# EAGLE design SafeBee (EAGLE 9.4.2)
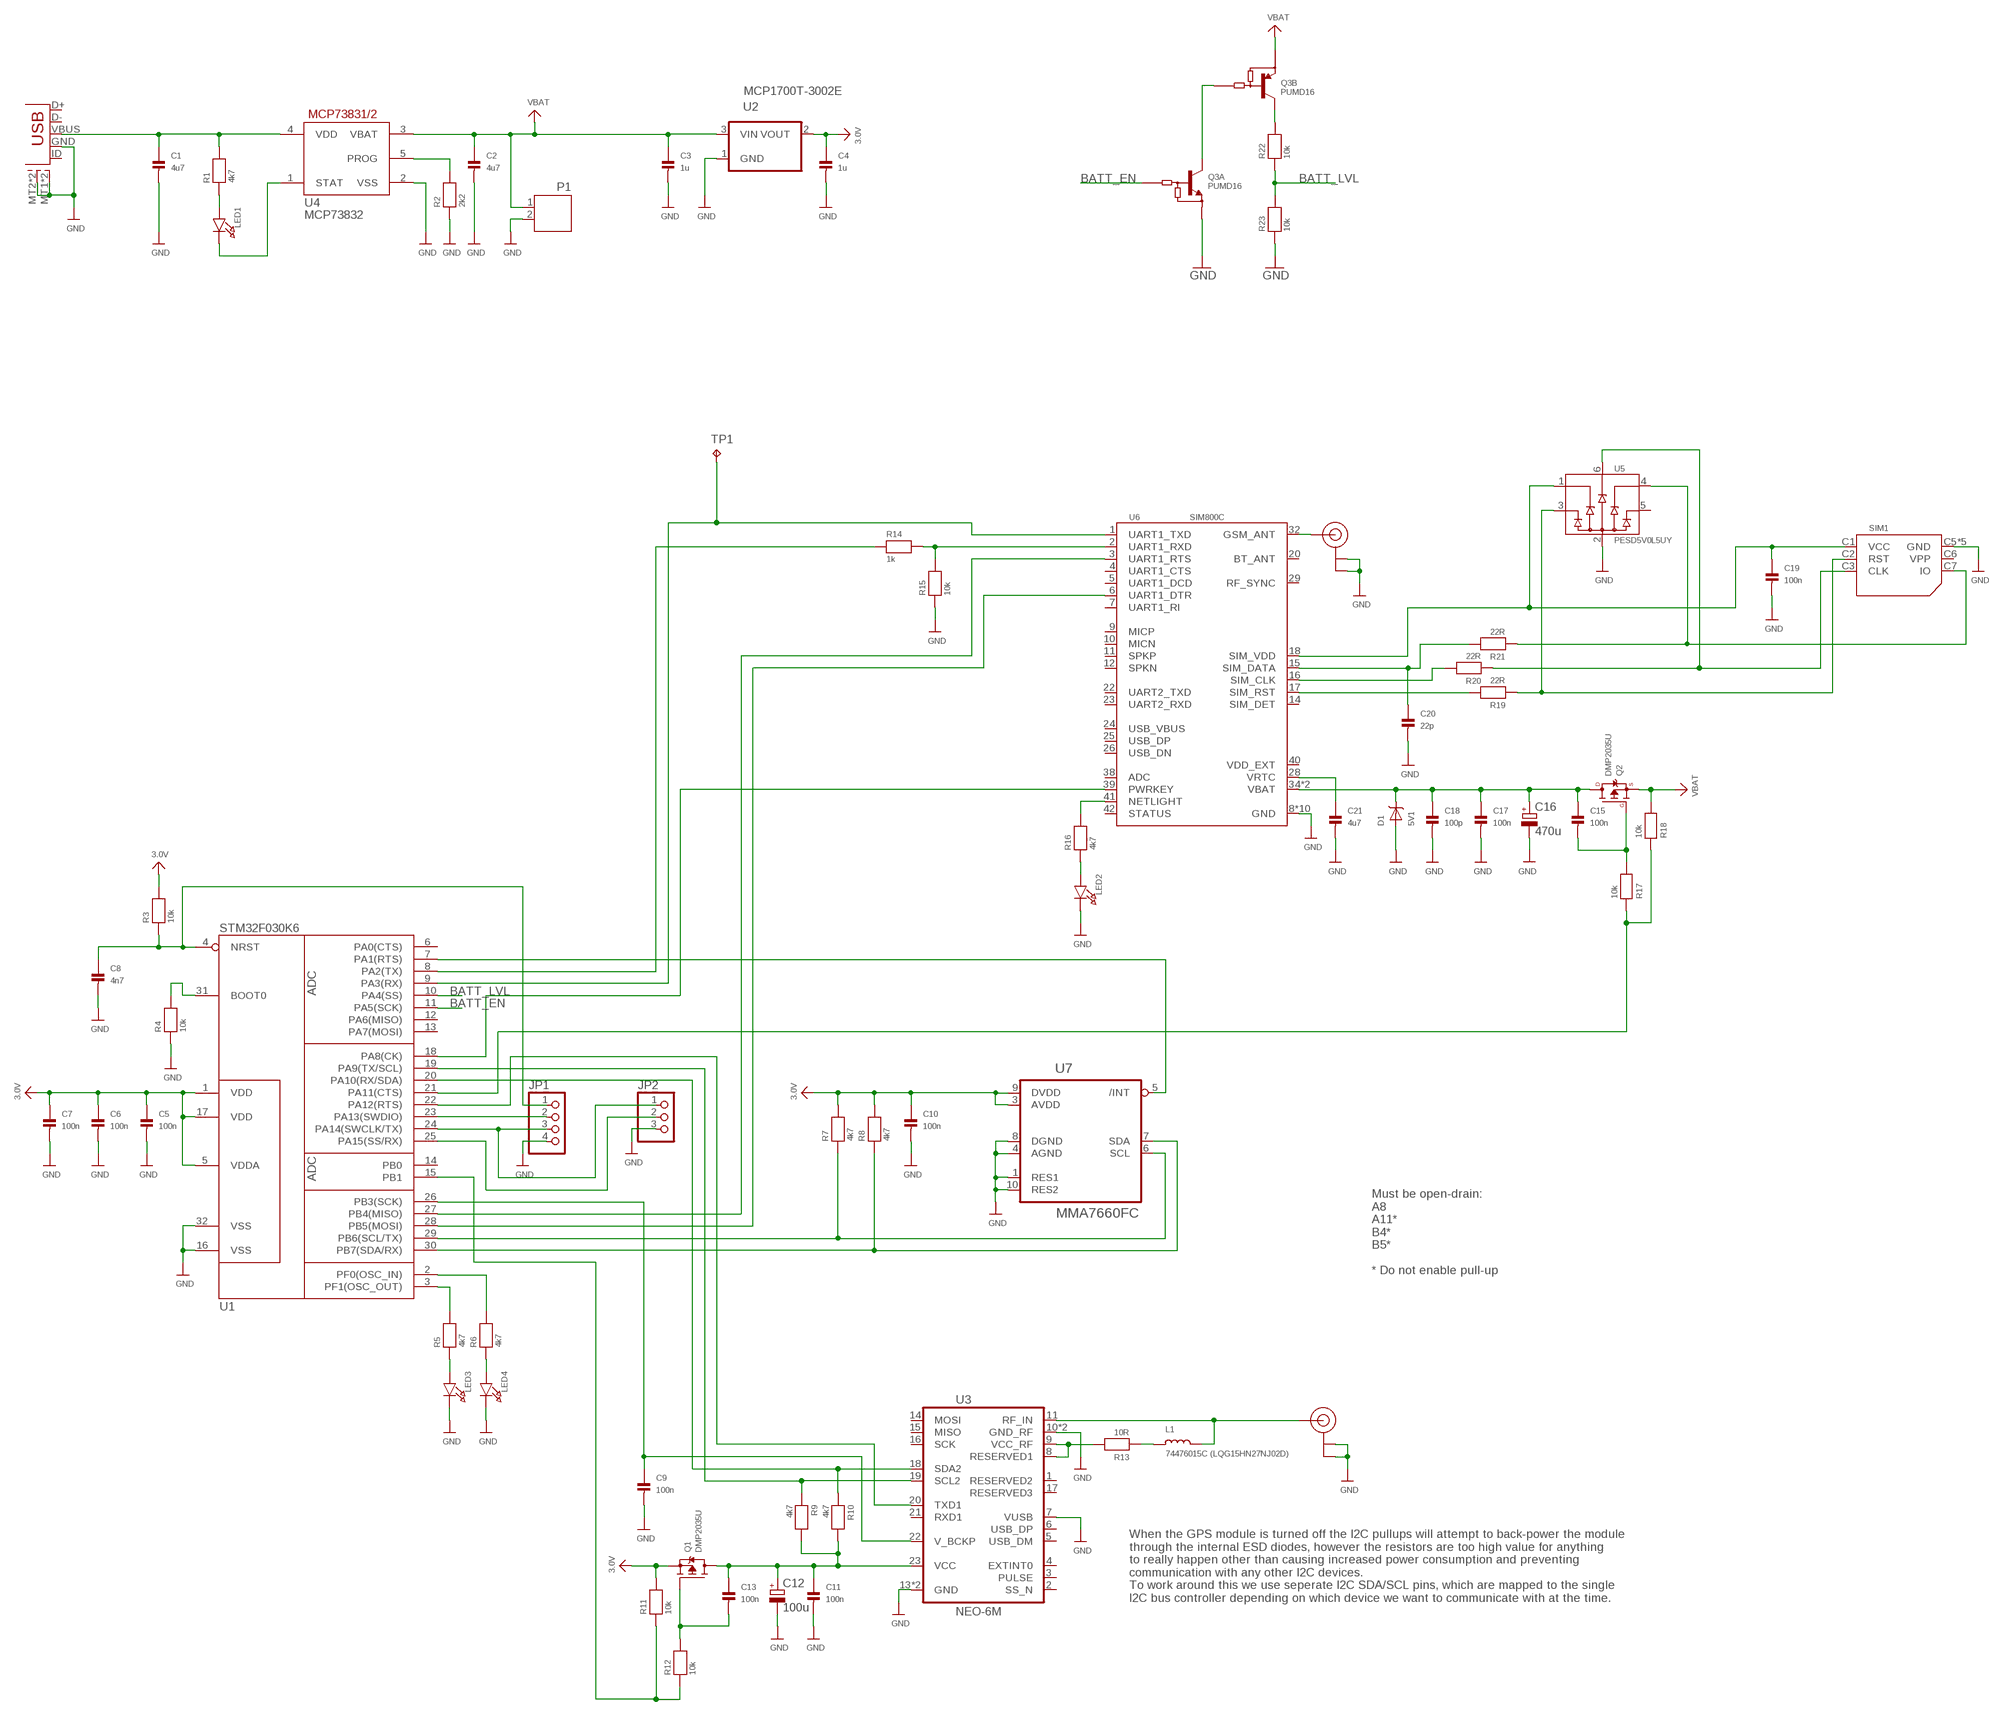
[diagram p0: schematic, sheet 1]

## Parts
C1  4u7  CAP_CERAMIC0805  [0805_NO_OUTLINE]
C2  4u7  CAP_CERAMIC0805  [0805_NO_OUTLINE]
C3  1u  CAP_CERAMIC0805  [0805_NO_OUTLINE]
C4  1u  CAP_CERAMIC0805  [0805_NO_OUTLINE]
C5  100n  CAP_CERAMIC0805  [0805_NO_OUTLINE]
C6  100n  CAP_CERAMIC0805  [0805_NO_OUTLINE]
C7  100n  CAP_CERAMIC0805  [0805_NO_OUTLINE]
C8  4n7  CAP_CERAMIC0805  [0805_NO_OUTLINE]
C9  100n  CAP_CERAMIC0805  [0805_NO_OUTLINE]
C10  100n  CAP_CERAMIC0805  [0805_NO_OUTLINE]
C11  100n  CAP_CERAMIC0805  [0805_NO_OUTLINE]
C12  100u  CPOL-EUE2.5-6  [E2,5-6]
C13  100n  CAP_CERAMIC0805  [0805_NO_OUTLINE]
C15  100n  CAP_CERAMIC0805  [0805_NO_OUTLINE]
C16  470u  CPOL-EUE2.5-6  [E2,5-6]
C17  100n  CAP_CERAMIC0805  [0805_NO_OUTLINE]
C18  100p  CAP_CERAMIC0805  [0805_NO_OUTLINE]
C19  100n  CAP_CERAMIC0805  [0805_NO_OUTLINE]
C20  22p  CAP_CERAMIC0805  [0805_NO_OUTLINE]
C21  4u7  CAP_CERAMIC0805  [0805_NO_OUTLINE]
D1  5V1  DIODE-ZENERSOD-123  [SOD-123]
JP1  PINHD-1X4  [1X04]
JP2  PINHD-1X3  [1X03]
L1  74476015C (LQG15HN27NJ02D)  INDUCTOR0805  [0805_NO_OUTLINE]
LED1  LED0603_NOOUTLINE  [CHIPLED_0603_NOOUTLINE]
LED2  LED0603_NOOUTLINE  [CHIPLED_0603_NOOUTLINE]
LED3  LED0603_NOOUTLINE  [CHIPLED_0603_NOOUTLINE]
LED4  LED0603_NOOUTLINE  [CHIPLED_0603_NOOUTLINE]
P1  JST-PH2  [JST-PH2]
Q1  DMP2035U  MOSFET-PWIDE  [SOT23-WIDE]
Q2  DMP2035U  MOSFET-PSOT-23-WIDE  [SOT-23-WIDE]
Q3  PUMD16  DUAL_NPNPNPDIGITALSOT-363  [SOT-363]
R1  4k7  RESISTOR0805_NO_OUTLINE  [0805_NO_OUTLINE]
R2  2k2  RESISTOR0805_NO_OUTLINE  [0805_NO_OUTLINE]
R3  10k  RESISTOR0805_NO_OUTLINE  [0805_NO_OUTLINE]
R4  10k  RESISTOR0805_NO_OUTLINE  [0805_NO_OUTLINE]
R5  4k7  RESISTOR0805_NO_OUTLINE  [0805_NO_OUTLINE]
R6  4k7  RESISTOR0805_NO_OUTLINE  [0805_NO_OUTLINE]
R7  4k7  RESISTOR0805_NO_OUTLINE  [0805_NO_OUTLINE]
R8  4k7  RESISTOR0805_NO_OUTLINE  [0805_NO_OUTLINE]
R9  4k7  RESISTOR0805_NO_OUTLINE  [0805_NO_OUTLINE]
R10  4k7  RESISTOR0805_NO_OUTLINE  [0805_NO_OUTLINE]
R11  10k  RESISTOR0805_NO_OUTLINE  [0805_NO_OUTLINE]
R12  10k  RESISTOR0805_NO_OUTLINE  [0805_NO_OUTLINE]
R13  10R  RESISTOR0805_NO_OUTLINE  [0805_NO_OUTLINE]
R14  1k  RESISTOR0805_NO_OUTLINE  [0805_NO_OUTLINE]
R15  10k  RESISTOR0805_NO_OUTLINE  [0805_NO_OUTLINE]
R16  4k7  RESISTOR0805_NO_OUTLINE  [0805_NO_OUTLINE]
R17  10k  RESISTOR0805_NO_OUTLINE  [0805_NO_OUTLINE]
R18  10k  RESISTOR0805_NO_OUTLINE  [0805_NO_OUTLINE]
R19  22R  RESISTOR0805_NO_OUTLINE  [0805_NO_OUTLINE]
R20  22R  RESISTOR0805_NO_OUTLINE  [0805_NO_OUTLINE]
R21  22R  RESISTOR0805_NO_OUTLINE  [0805_NO_OUTLINE]
R22  10k  RESISTOR0805_NO_OUTLINE  [0805_NO_OUTLINE]
R23  10k  RESISTOR0805_NO_OUTLINE  [0805_NO_OUTLINE]
SIM1  SIMCARDSOCKET  [SIM_SOCKET1]
TP1  TPTP10R  [TP10R]
U1  STM32F030K6  [TQFP32-08]
U2  MCP1700T-3002E  MCP1700T-2502E/TTWIDE_PAD  [SOT-23]
U3  NEO-6M  [NEO-6M]
U4  MCP73831/OT  [SOT23-5L]
U5  PESD5V0L5UY  ESD5DIODEARRAYSOT-363  [SOT-363]
U6  SIM800C  [SIM800C]
U7  MMA7660FC  [DFN_3X3_10]
U$1  USB-MICROBSAFEBEE  [USB-MICROB_SAFEBEE]
U$47  U.FL  [U.FL]
U$55  U.FL  [U.FL]

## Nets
3.0V: C4.1 C5.1 C6.1 C7.1 C10.1 Q1.2(S) R3.2 R7.2 R8.2 R11.2 U1.1(VDD) U1.5(VDDA) U1.17(VDD) U2.2(VOUT) U7.3(AVDD) U7.9(DVDD)
BATT_EN: Q3.2(A:B) U1.11(PA5(SCK))
BATT_LVL: R22.1 R23.2 U1.10(PA4(SS))
GND: C1.2 C2.2 C3.2 C4.2 C5.2 C6.2 C7.2 C8.2 C9.2 C10.2 C11.2 C12.- C16.- C17.2 C18.2 C19.2 C20.2 C21.2 D1.A JP1.4 JP2.3 LED2.C LED3.C LED4.C P1.2 Q3.1(A:E) R2.1 R4.1 R15.1 R23.1 SIM1.C5(GND) SIM1.GND1(GND) SIM1.GND2(GND) SIM1.GND3(GND) SIM1.GND4(GND) U1.16(VSS) U1.32(VSS) U2.1(GND) U3.7(VUSB) U3.10(GND_RF) U3.12(GND_RF) U3.13(GND) U3.24(GND) U4.2(VSS) U5.2(GND) U6.8(GND) U6.13(GND) U6.19(GND) U6.21(GND) U6.27(GND) U6.30(GND) U6.31(GND) U6.33(GND) U6.36(GND) U6.37(GND) U7.1(RES1) U7.4(AGND) U7.8(DGND) U7.10(RES2) U$1.GND U$1.MT1(SHEILD1) U$1.MT2(SHEILD2) U$1.MT3(SHEILD1) U$1.MT4(SHEILD2) U$47.1(GND) U$47.2(GND) U$55.1(GND) U$55.2(GND)
N$1: U1.22(PA12(RTS)) U3.20(TXD1)
N$2: LED1.A R1.1
N$3: R19.1 SIM1.C2(RST) U5.3(IO2)
N$4: C9.1 U1.26(PB3(SCK)) U3.22(V_BCKP)
N$5: R2.2 U4.5(PROG)
N$7: JP1.2 U1.23(PA13(SWDIO))
N$8: JP1.3 JP2.1 U1.24(PA14(SWCLK/TX))
N$9: L1.1 R13.1
N$10: C8.1 JP1.1 R3.1 U1.4(NRST)
N$11: U1.7(PA1(RTS)) U7.5(/INT)
N$12: Q3.5(B:B) Q3.6(A:C)
N$13: C19.1 SIM1.C1(VCC) U5.1(IO1) U6.18(SIM_VDD)
N$14: JP2.2 U1.25(PA15(SS/RX))
N$15: R9.1 U1.19(PA9(TX/SCL)) U3.19(SCL2)
N$16: R10.1 U1.20(PA10(RX/SDA)) U3.18(SDA2)
N$17: Q3.3(B:C) R22.2
N$18: R20.1 SIM1.C3(CLK) U5.6(IO5)
N$19: L1.2 U3.11(RF_IN) U$47.3(SIGNAL)
N$21: R13.2 U3.8(RESERVED1) U3.9(VCC_RF)
N$23: C20.1 R21.2 U6.15(SIM_DATA)
N$24: U6.32(GSM_ANT) U$55.3(SIGNAL)
N$25: C15.1 C16.+ C17.1 C18.1 D1.C Q2.3(D) U6.34(VBAT) U6.35(VBAT)
N$26: U1.27(PB4(MISO)) U6.3(UART1_RTS)
N$27: R14.1 U1.8(PA2(TX))
N$28: U1.28(PB5(MOSI)) U6.6(UART1_DTR)
N$29: R16.2 U6.41(NETLIGHT)
N$30: R5.2 U1.3(PF1(OSC_OUT))
N$31: TP1.TP U1.9(PA3(RX)) U6.1(UART1_TXD)
N$32: R4.2 U1.31(BOOT0)
N$33: LED2.A R16.1
N$34: R21.1 SIM1.C7(IO) U5.4(IO3)
N$35: C1.1 R1.2 U4.4(VDD) U$1.VBUS
N$36: R8.1 U1.30(PB7(SDA/RX)) U7.7(SDA)
N$37: R7.1 U1.29(PB6(SCL/TX)) U7.6(SCL)
N$38: R6.2 U1.2(PF0(OSC_IN))
N$39: C21.1 U6.28(VRTC)
N$40: R17.1 R18.1 U1.21(PA11(CTS))
N$41: LED1.C U4.1(STAT)
N$42: C11.1 C12.+ C13.1 Q1.3(D) R9.2 R10.2 U3.23(VCC)
N$44: U1.18(PA8(CK)) U6.39(PWRKEY)
N$47: LED3.A R5.1
N$48: R14.2 R15.2 U6.2(UART1_RXD)
N$49: LED4.A R6.1
N$50: C15.2 Q2.1(G) R17.2
N$53: R11.1 R12.1 U1.15(PB1)
N$54: C13.2 Q1.1(G) R12.2
N$56: R20.2 U6.16(SIM_CLK)
N$57: R19.2 U6.17(SIM_RST)
VBAT: C2.1 C3.1 P1.1 Q2.2(S) Q3.4(B:E) R18.2 U2.3(VIN) U4.3(VBAT)
Unconnected: SIM1.C6(VPP) U1.6(PA0(CTS)) U1.12(PA6(MISO)) U1.13(PA7(MOSI)) U1.14(PB0) U3.1(RESERVED2) U3.2(SS_N) U3.3(PULSE) U3.4(EXTINT0) U3.5(USB_DM) U3.6(USB_DP) U3.14(MOSI) U3.15(MISO) U3.16(SCK) U3.17(RESERVED3) U3.21(RXD1) U5.5(IO4) U6.4(UART1_CTS) U6.5(UART1_DCD) U6.7(UART1_RI) U6.9(MICP) U6.10(MICN) U6.11(SPKP) U6.12(SPKN) U6.14(SIM_DET) U6.20(BT_ANT) U6.22(UART2_TXD) U6.23(UART2_RXD) U6.24(USB_VBUS) U6.25(USB_DP) U6.26(USB_DN) U6.29(RF_SYNC) U6.38(ADC) U6.40(VDD_EXT) U6.42(STATUS) U$1.D+ U$1.D- U$1.ID

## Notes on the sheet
- MCP73832
- Must be open-drain:
  A8
  A11*
  B4*
  B5*
  
  * Do not enable pull-up
- When the GPS module is turned off the I2C pullups will attempt to back-power the module
  through the internal ESD diodes, however the resistors are too high value for anything
  to really happen other than causing increased power consumption and preventing
  communication with any other I2C devices.
  To work around this we use seperate I2C SDA/SCL pins, which are mapped to the single
  I2C bus controller depending on which device we want to communicate with at the time.

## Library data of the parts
C1-C11 C13 C15 C17-C21 = zak:CAP_CERAMIC
C12 C16 = resistor:CPOL-EU: POLARIZED CAPACITOR, European symbol
D1 = zak:DIODE-ZENER
JP1 = pinhead:PINHD-1X4: PIN HEADER
JP2 = pinhead:PINHD-1X3: PIN HEADER
L1 = zak:INDUCTOR
LED1-LED4 = microbuilder:LED: LED
P1 = jst-ph:JST-PH2
Q1 = microbuilder:MOSFET-P: P-Channel Mosfet LEGEND VDS: Voltage Drain-Source ID: Drain Current RDS(ON): Drain-Source On-State Resistance VGS(TH): Gate-Source Threshold Voltage CISS: Drain-Source Input Capacitance SOT-23 Name VDS ID RDS(ON) VGS(TH) CISS Order Number IRLML5103 30V 760mA 600 mOhm -- 75pF @ 25V Digikey: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
Q2 = zak:MOSFET-P
Q3 = zak:DUAL_NPNPNPDIGITAL
R1-R23 = zak:RESISTOR
SIM1 = zak:SIMCARDSOCKET
TP1 = testpad:TP: Test pad
U1 = zak:STM32F030K6
U2 = zak:MCP1700T-2502E/TT: Low Quiescent Current LDO
U3 = zak:NEO-6M
U4 = adafruit:MCP73831: MCP73831/2 Miniature Single-Cell, Fully Integrated Li-Ion, Li-Polymer Charge Management Controllers. Nice and small simple lipoly charge controller, with adjustable current and status output (LED) http://www.ladyada.net/library/pcb/eaglelibrary.html
U5 = zak:ESD5DIODEARRAY
U6 = zak:SIM800C
U7 = zak:MMA7660FC
U$1 = zak:USB-MICROB
U$47 U$55 = microbuilder:U.FL: U.FL Antenna Connector

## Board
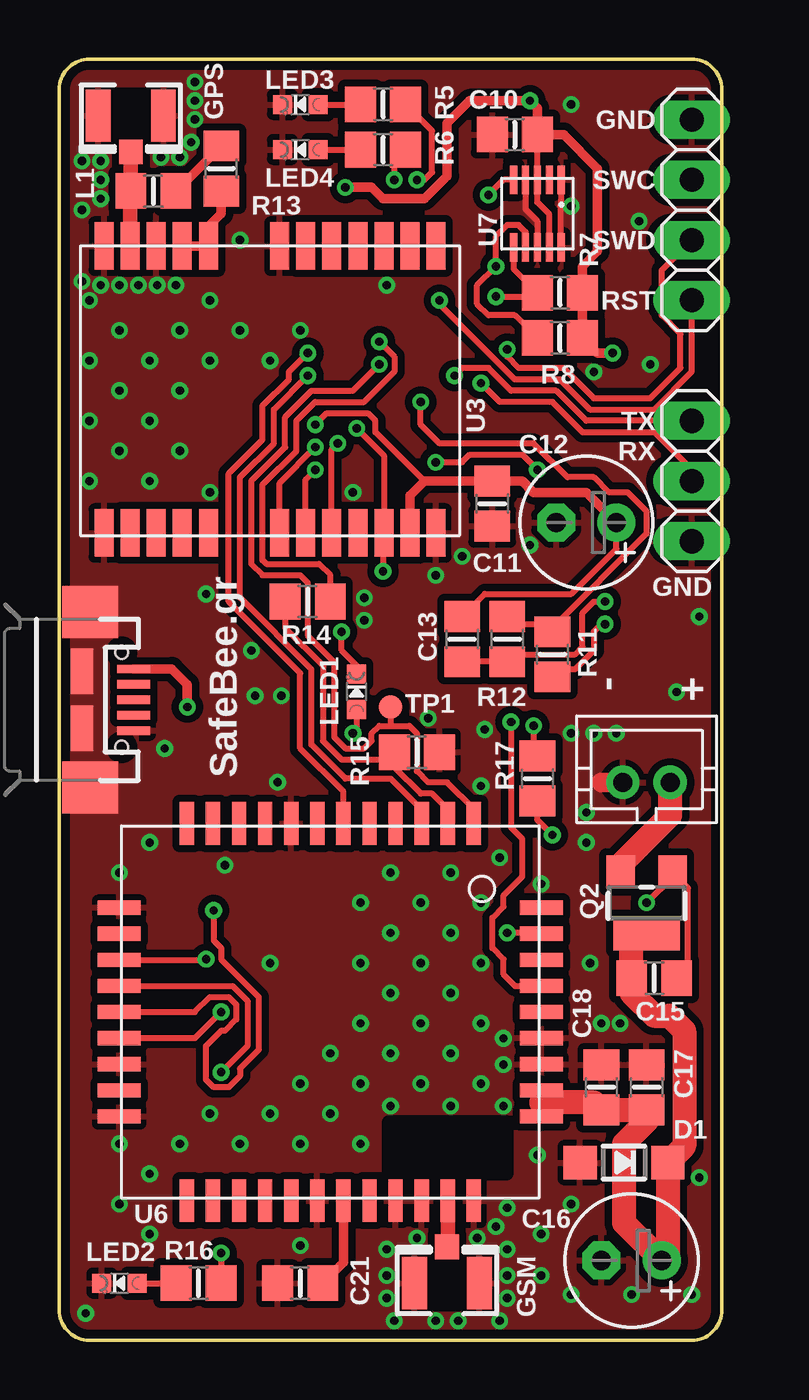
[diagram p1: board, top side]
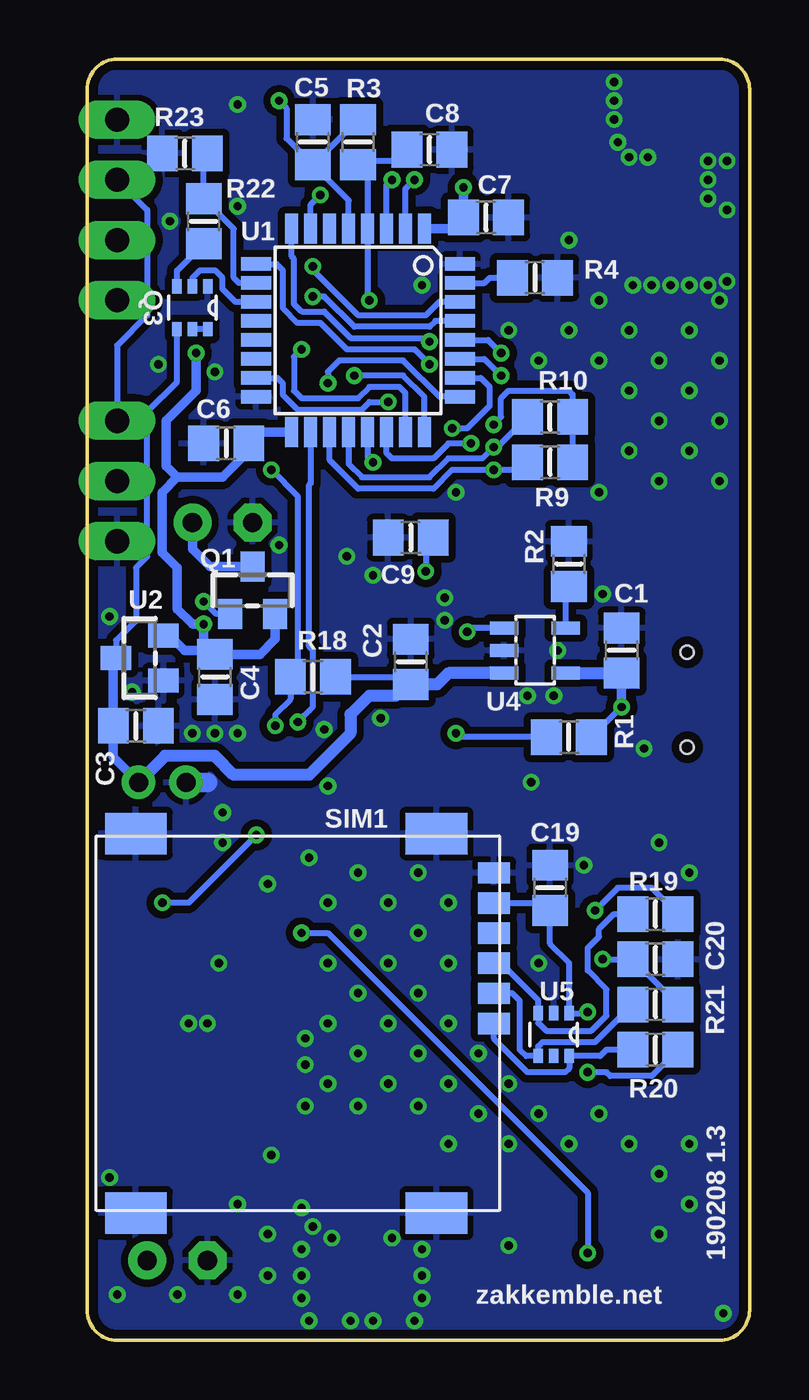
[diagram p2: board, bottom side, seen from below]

Size 27.94 x 54 mm. Coordinates in mm from the lower left corner, seen from the top.
Outline: 26.67,54 arc-90 27.94,52.73 27.94,1.27 arc-90 26.67,0 1.27,0 arc-90 0,1.27 0,52.73 arc-90 1.27,54 26.67,54
Copper layers (1*16): Top 0.0356mm / dielectric 1.5011mm / Bottom 0.0356mm
Design rules "LaenPCBOrder *": minimum track width 6mil, minimum drill 13mil, track to track 6mil, track to pad 6mil, pad to pad 6mil, via to via 6mil, smd to smd 6mil, copper to edge 15mil, drill to drill 6mil, minimum pad ring 12mil, minimum via ring 7mil, stop-mask expansion 2.5mil, vias tented up to drill 24mil, thermal gap 10mil

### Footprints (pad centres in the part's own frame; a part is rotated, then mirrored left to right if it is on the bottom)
0805_NO_OUTLINE = smd 1.3 x 1.5: 1 -0.95,0; 2 0.95,0
E2,5-6 = drill 0.813 pad 1.6: + -1.27,0 | drill 0.813 pad 1.6 octagon: - 1.27,0
SOD-123 = smd 1.4 x 1.4: A 1.85,0; C -1.85,0
1X04 = drill 1.016 long: 1 -3.81,0; 2 -1.27,0; 3 1.27,0; 4 3.81,0
1X03 = drill 1.016 long: 1 -2.54,0; 2 0,0; 3 2.54,0
CHIPLED_0603_NOOUTLINE = smd 0.8 x 0.8: A 0,-0.75; C 0,0.75
JST-PH2 = drill 0.8: 1 1,0; 2 -1,0
SOT23-WIDE = smd 1 x 1.27: 1 -0.95,-1; 2 0.95,-1; 3 0,1
SOT-23-WIDE = smd 1.2 x 1.4: 1 -1.1,-1.3; 2 1.1,-1.3 | smd 2.8 x 1.4: 3 0,1.3
SOT-363 = smd 0.6 x 0.4: 1 -0.9,0.65; 2 -0.9,0; 3 -0.9,-0.65; 4 0.9,-0.65; 5 0.9,0; 6 0.9,0.65
SIM_SOCKET1 = smd 0.9 x 1.35: C1 -5.07,8.275; C2 -2.53,8.275; C3 0.01,8.275; C5 -6.34,8.275; C6 -3.8,8.275; C7 -1.26,8.275 | smd 1.75 x 2.6: GND1 -8,5.85; GND2 -8,-6.83; GND3 8,5.85; GND4 8,-6.83
TP10R = smd 1 x 1: TP 0,0
TQFP32-08 = smd 1.27 x 0.559: 1 -4.293,2.8; 2 -4.293,2; 3 -4.293,1.2; 4 -4.293,0.4; 5 -4.293,-0.4; 6 -4.293,-1.2; 7 -4.293,-2; 8 -4.293,-2.8; 17 4.293,-2.8; 18 4.293,-2; 19 4.293,-1.2; 20 4.293,-0.4; 21 4.293,0.4; 22 4.293,1.2; 23 4.293,2; 24 4.293,2.8 | smd 0.559 x 1.27: 9 -2.8,-4.293; 10 -2,-4.293; 11 -1.2,-4.293; 12 -0.4,-4.293; 13 0.4,-4.293; 14 1.2,-4.293; 15 2,-4.293; 16 2.8,-4.293; 25 2.8,4.293; 26 2,4.293; 27 1.2,4.293; 28 0.4,4.293; 29 -0.4,4.293; 30 -1.2,4.293; 31 -2,4.293; 32 -2.8,4.293
SOT-23 = smd 1 x 1.27: 1 -0.95,-1; 2 0.95,-1; 3 0,1
NEO-6M = smd 2 x 0.8: 1 6.1,-7; 2 6.1,-5.9; 3 6.1,-4.8; 4 6.1,-3.7; 5 6.1,-2.6; 6 6.1,-1.5; 7 6.1,-0.4; 8 6.1,2.6; 9 6.1,3.7; 10 6.1,4.8; 11 6.1,5.9; 12 6.1,7; 13 -6,7; 14 -6,5.9; 15 -6,4.8; 16 -6,3.7; 17 -6,2.6; 18 -6,-0.4; 19 -6,-1.5; 20 -6,-2.6; 21 -6,-3.7; 22 -6,-4.8; 23 -6,-5.9; 24 -6,-7
SOT23-5L = smd 0.55 x 1.2: 1 -0.95,-1.3; 2 0,-1.3; 3 0.95,-1.3; 4 0.95,1.3; 5 -0.95,1.3
SIM800C = smd 1.8 x 0.6: 1 -7.95,6.05; 2 -7.95,4.95; 3 -7.95,3.85; 4 -7.95,2.75; 5 -7.95,1.65; 6 -7.95,0.55; 7 -7.95,-0.55; 8 -7.95,-1.65; 9 -7.95,-2.75; 10 -7.95,-3.85; 11 -7.95,-4.95; 12 -7.95,-6.05; 22 7.95,-6.05; 23 7.95,-4.95; 24 7.95,-3.85; 25 7.95,-2.75; 26 7.95,-1.65; 27 7.95,-0.55; 28 7.95,0.55; 29 7.95,1.65; 30 7.95,2.75; 31 7.95,3.85; 32 7.95,4.95; 33 7.95,6.05 | smd 0.6 x 1.8: 13 -4.4,-8.9; 14 -3.3,-8.9; 15 -2.2,-8.9; 16 -1.1,-8.9; 17 0,-8.9; 18 1.1,-8.9; 19 2.2,-8.9; 20 3.3,-8.9; 21 4.4,-8.9; 34 4.4,8.9; 35 3.3,8.9; 36 2.2,8.9; 37 1.1,8.9; 38 0,8.9; 39 -1.1,8.9; 40 -2.2,8.9; 41 -3.3,8.9; 42 -4.4,8.9
DFN_3X3_10 = smd 1.205 x 0.3: 1 -1.43,1; 2 -1.43,0.5; 3 -1.43,0; 4 -1.43,-0.5; 5 -1.43,-1; 6 1.43,-1; 7 1.43,-0.5; 8 1.43,0; 9 1.43,0.5; 10 1.43,1
USB-MICROB_SAFEBEE = smd 0.35 x 1.4: D+ 0,2.65; D- -0.65,2.65; GND 1.3,2.65; ID 0.65,2.65; VBUS -1.3,2.65 | smd 2.2 x 2.35: MT1 -3.7,0.825; MT2 3.7,0.825 | smd 1.9 x 0.95: MT3 -1.2,0.475; MT4 1.2,0.475 | hole 0.55: -2,2.15; 2,2.15
U.FL = smd 2.2 x 1.05: 1 0,1.375; 2 0,-1.375 | smd 1.05 x 1: 3 1.525,0

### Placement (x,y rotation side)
C1  5.4,29.08 90 bottom
C2  14.29,28.6 90 bottom
C3  25.88,25.9 0 bottom
C4  22.54,27.96 270 bottom
C5  18.41,50.51 90 bottom
C6  22.07,37.81 180 bottom
C7  11.11,47.33 0 bottom
C8  13.49,50.19 0 bottom
C9  14.29,33.84 180 bottom
C10  19.21,50.82 180 top
C11  18.26,35.27 270 top
C12  22.23,34.47 180 top
C13  16.99,29.55 270 top
C15  25.08,15.27 0 top
C16  24.13,3.36 180 top
C17  24.77,10.66 90 top
C18  22.86,10.66 90 top
C19  8.41,19.07 90 bottom
C20  3.97,16.06 0 bottom
C21  10.16,2.41 180 top
D1  23.81,7.49 180 top
JP1  26.67,47.65 90 top
JP2  26.67,36.22 270 top
L1  3.97,48.44 180 top
LED1  12.54,27.33 0 top
LED2  2.54,2.41 90 top
LED3  10.16,52.09 90 top
LED4  10.16,50.19 90 top
P1  24.77,23.52 0 top
Q1  20.95,31.62 0 bottom
Q2  24.77,18.44 180 top
Q3  23.5,43.52 270 bottom
R1  7.62,25.43 0 bottom
R2  7.62,32.73 270 bottom
R3  16.51,50.51 90 bottom
R4  9.05,44.79 180 bottom
R5  13.65,52.09 0 top
R6  13.65,50.19 0 top
R7  21.11,44.16 0 top
R8  21.11,42.25 0 top
R9  8.41,37.01 0 bottom
R10  8.41,38.92 0 bottom
R11  20.8,28.92 270 top
R12  18.89,29.55 270 top
R13  6.83,49.4 270 top
R14  10.48,31.14 180 top
R15  15.08,24.79 180 top
R16  5.87,2.41 0 top
R17  20.16,23.68 270 top
R18  18.41,27.96 0 bottom
R19  3.97,17.96 0 bottom
R20  3.97,12.25 0 bottom
R21  3.97,14.15 0 bottom
R22  23.02,47.17 270 bottom
R23  23.81,50.03 0 bottom
SIM1  19.05,13.36 270 bottom
TP1  13.97,26.7 0 top
U1  16.51,42.57 270 bottom
U2  25.72,28.76 90 bottom
U3  8.89,40.03 90 top
U4  9.05,29.08 270 bottom
U5  8.26,12.88 270 bottom
U6  11.43,13.84 270 top
U7  20.16,47.49 270 top
U$1  0.48,27 270 top
U$47  3.02,51.62 270 top
U$55  16.35,2.41 90 top

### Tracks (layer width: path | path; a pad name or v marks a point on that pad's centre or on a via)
3.0V  (via drill 0.35)
  Top 0.254: U7.9 20.66,47.47 20.16,47.97 U7.3 20.16,50.66 20.32,50.82 | R11.2 21.11,28.28 21.75,28.28 22.54,29.08 22.54,29.87 22.86,30.19 v23.02,30.19
  Top 0.406: v12.06,48.6 13.18,48.6 13.65,48.13 15.4,48.13 16.35,49.08 16.35,51.3 17.3,52.25 v19.84,52.25 20.16,51.94 C10.1 20.16,50.67 20.32,50.82 21.27,50.82 22.7,49.4 22.7,45.9 22.07,45.27 R7.2 R8.2 22.7,41.62 v23.34,41.62
  Bottom 0.254: U1.5 16.91,48.05 C5.1 | C5.1 R3.2 | C5.1 19.53,50.67 19.53,51.94 v19.84,52.25
  Bottom 0.406: v12.06,48.6 C7.1 12.53,46.86 U1.1 | 24.13,36.38 22.23,36.38 21.12,37.49 C6.1 20.65,38.28 U1.17 | 24.13,36.38 24.61,36.85 24.61,38.76 23.34,40.03 v23.34,41.62 | Q1.2 20,29.55 20.64,28.92 | 20.64,28.92 | 24.77,29.44 U2.2 24.45,29.71 23.81,29.08 22.7,29.08 | 24.13,36.38 24.77,35.74 24.77,33.2 24.13,32.57 24.13,30.82 23.5,30.19 v23.02,30.19 23.02,29.4 22.7,29.08 | 20.64,28.92 C4.1 | C4.1 | 22.7,29.08 C4.1
BATT_EN
  Bottom 0.254: Q3.2 23.5,44.79 23.18,45.11 22.54,45.11 22.23,44.79 22.23,44.32 21.68,43.77 U1.11
BATT_LVL
  Bottom 0.254: U1.10 21.53,44.57 21.75,44.79 21.75,46.85 R22.1 23.02,49.88 R23.2
GND  (via drill 0.35)
  Top 0.254: U7.1 21.16,47.86 21.11,47.81 21.27,47.81 | 21.27,47.81 v21.59,47.81 | U7.10 21.16,47.7 21.27,47.81 | U7.8 20.16,47.17 19.66,47.67 U7.4
  Top 0.813: P1.2 22.86,23.52
  Bottom 0.813: P1.2 22.86,23.52
  other vias: 4.45,24.95 8.26,27.17 15.88,32.25 18.73,12.73 18.73,11.61 24.92,41.14 12.86,31.3 22.54,40.82 24.45,47.17 21.59,52.09 5.71,53.05 5.71,52.25 5.71,51.46 1.75,49.71 0.95,49.71 1.75,48.92 1.75,48.13 0.95,47.65 0.95,44.63 1.75,44.47 2.54,44.47 3.33,44.47 4.13,44.47 4.92,44.47 4.29,49.87 5.08,49.87 5.56,50.51 17.62,4.31 15.08,4.31 18.41,4.79 18.89,5.58 18.89,3.83 18.89,2.72 18.89,1.77 18.57,0.82 15.88,0.82 16.83,0.82 16.99,33.04 19.84,33.52 26.99,30.5 20.16,7.8 21.59,5.74 26.67,1.93 17.94,25.74 17.78,23.36 22.54,25.58 23.5,25.58 21.59,25.58 13.81,44.47 2.54,42.57 5.08,42.57 6.35,41.3 3.81,41.3 2.54,40.03 5.08,40.03 3.81,38.76 2.54,37.49 3.81,36.22 5.08,37.49 7.62,42.57 8.89,41.3 10.16,42.57 1.27,41.3 1.27,38.76 1.27,36.22 6.35,43.84 1.27,43.84 6.35,35.74 7.62,46.38 10.16,3.99 13.81,1.77 14.13,0.82 12.86,30.35 6.19,31.46 20.32,4.47 20.32,2.72 21.59,1.93 8.1,29.08 15.56,26.22 18.57,20.35 17.78,18.44 12.38,35.74 22.86,13.36 22.23,20.98 20.32,19.23 9.21,23.52 6.99,20.03 8.89,15.9 13.97,12.09 12.7,10.82 12.7,8.28 7.62,8.28 5.08,8.28 10.16,8.28 11.43,9.55 3.81,7.01 16.51,12.09 15.24,13.36 15.24,10.82 17.78,10.82 17.78,13.36 17.78,15.9 26.99,6.85 22.38,15.9 24.13,1.93 23.65,13.36 16.51,14.63 13.81,2.72 13.81,3.83 2.54,5.74 3.81,4.47 3.81,20.98 26.04,27.33 12.7,15.9 11.43,12.09 10.16,10.82 6.35,9.55 8.89,9.55 2.54,8.28 1.11,1.14 16.51,17.17 16.51,19.71 22.23,22.25 15.24,15.9 13.97,14.63 13.97,17.17 15.24,18.44 13.97,19.71 12.7,18.44 12.7,13.36 2.54,19.71 16.51,9.87 13.97,9.87 18.73,9.87 9.37,27.17
  pour Top (isolate 0.305, rank 6): 0,0 0,54 27.94,54 27.94,0
  pour Bottom (isolate 0.305, rank 6): 0,0 0,54 27.94,54 27.94,0
  pour Top (isolate 0.305, rank 5, no thermals): 0,32.25 3.33,32.25 3.33,21.77 0,21.77
N$1  (via drill 0.35)
  Top 0.254: U3.20 11.49,37.55 v11.75,37.81
  Bottom 0.254: v11.75,37.81 12.7,37.81 13.34,37.17 15.08,37.17 15.31,37.4 U1.22
N$2  (via drill 0.35)
  Top 0.254: LED1.A 12.54,25.74 v12.38,25.58
  Bottom 0.254: R1.1 12.22,25.43 v12.38,25.58
N$3
  Bottom 0.254: SIM1.C2 10.47,15.89 8.9,14.33 U5.3 8.9,13.38 8.57,13.04 6.67,13.04 6.35,13.36 6.03,13.68 6.03,14.79 6.83,15.58 6.83,16.54 6.35,17.01 6.35,17.33 5.71,17.96 R19.1
N$4  (via drill 0.35)
  Top 0.254: v12.54,38.44 13.69,37.29 U3.22 13.65,33.99 v13.65,32.41
  Bottom 0.254: U1.26 11.34,40.57 10.95,40.19 10.95,39.39 11.91,38.44 v12.54,38.44 | C9.1 13.65,33.52 v13.65,32.41
N$5
  Bottom 0.254: U4.5 7.75,31.65 R2.2
N$7  (via drill 0.35)
  Top 0.254: v18.89,41.78 18.89,41.46 19.37,40.98 21.27,40.98 22.54,39.71 24.13,39.71 24.29,39.71 24.92,39.71 26.19,40.98 26.19,42.41 25.4,43.2 25.4,45.11 JP1.2
  Bottom 0.254: U1.23 14.51,39.93 14.76,40.19 16.03,40.19 16.51,39.71 18.89,39.71 19.21,40.03 19.21,41.46 v18.89,41.78
N$8  (via drill 0.35)
  Top 0.254: JP2.1 22.23,38.76 20.95,40.03 19.05,40.03 18.1,40.98 16.99,40.98 v16.67,40.66
  Bottom 0.254: U1.24 13.71,39.77 14.61,40.66 v16.67,40.66 | JP1.3 25.4,47.65 25.4,43.2 26.67,41.93 JP2.1
N$9
  Top 0.406: L1.1 R13.1
N$10  (via drill 0.35)
  Top 0.254: v16.03,43.84 16.03,43.68 19.21,40.51 21.11,40.51 22.38,39.24 25.08,39.24 26.67,40.82 JP1.1
  Bottom 0.254: C8.1 14.44,49.72 14.45,49.71 16.35,49.71 R3.1 16.11,49.16 U1.4 16.11,43.92 v16.03,43.84
N$11  (via drill 0.35)
  Top 0.254: U7.5 18.73,48.92 v18.1,48.28
  Bottom 0.254: U1.7 18.51,47.87 v18.1,48.28
N$12
  Bottom 0.254: Q3.6 Q3.5
N$13  (via drill 0.35)
  Top 0.254: U6.18 5.73,12.74 v6.83,13.84
  Bottom 0.254: v6.83,13.84 6.88,13.78 U5.1 7.61,15.9 8.41,16.71 C19.1 8.72,18.43 SIM1.C1
N$14  (via drill 0.35)
  Top 0.254: v17.78,40.35 18.57,39.55 20.8,39.55 22.07,38.28 25.08,38.28 26.67,36.7 JP2.2
  Bottom 0.254: U1.25 13.07,39.77 14.61,41.3 17.3,41.3 17.78,40.82 v17.78,40.35
N$15  (via drill 0.35)
  Top 0.254: v10.79,36.7 10.39,36.29 U3.19
  Bottom 0.254: U1.19 17.71,37.1 16.51,35.9 13.34,35.9 12.54,36.7 v10.79,36.7 9.68,36.7 R9.1
N$16  (via drill 0.35)
  Top 0.254: v10.79,37.65 9.29,36.14 U3.18
  Bottom 0.254: U1.20 16.91,36.94 16.35,36.38 13.49,36.38 12.7,37.17 11.27,37.17 v10.79,37.65 10.63,37.65 R10.1
N$17
  Bottom 0.254: Q3.3 24.14,45.1 R22.2
N$18
  Bottom 0.254: R20.1 6.03,12.25 6.3,11.98 U5.6 7.61,11.47 7.78,11.3 9.37,11.3 10.78,12.71 SIM1.C3
N$19
  Top 0.61: U3.11 2.99,48.41 L1.2 U$47.3
N$21
  Top 0.406: R13.2 6.83,47.49 6.29,46.95 U3.8 U3.9
N$23  (via drill 0.35)
  Top 0.254: U6.15 6.17,16.04 v6.19,16.06
  Bottom 0.254: R21.2 C20.1 v6.19,16.06
N$24
  Top 0.61: U6.32 16.38,4.06 U$55.3
N$25
  Top 0.61: U6.35 20.33,10.03 U6.34
  Top 1.016: Q2.3 24.26,17.14 24.13,17.01 C15.1 24.13,14.63 25.08,13.68 25.72,13.68 26.35,13.04 26.35,8.18 D1.C 25.66,3.62 C16.+ 23.81,4.95 23.81,8.28 24.77,9.23 C17.1 C18.1 22.55,10.03 20.33,10.03
N$26  (via drill 0.35)
  Top 0.254: U6.3 15.28,22.37 13.97,23.68 12.7,23.68 12.38,23.68 12.06,23.68 10.64,25.11 10.64,28.28 7.62,31.3 7.62,36.38 9.05,37.81 9.05,39.24 v10.48,40.66
  Bottom 0.254: U1.27 11.18,41.37 v10.48,40.66
N$27  (via drill 0.35)
  Top 0.254: v13.49,42.09 14.13,41.46 14.13,40.82 12.86,39.55 10.79,39.55 10,38.76 10,37.49 8.57,36.06 8.57,32.89 8.73,32.73 10.95,32.73 11.43,32.25 R14.1
  Bottom 0.254: U1.8 19.31,45.69 19.21,45.59 19.21,43.68 18.89,43.36 17.94,43.36 16.83,42.25 13.65,42.25 v13.49,42.09
N$28  (via drill 0.35)
  Top 0.254: v10.48,41.62 9.68,40.82 9.68,40.51 8.57,39.39 8.57,37.97 7.14,36.54 7.14,31.14 10.16,28.12 10.16,24.95 11.98,23.13 U6.6
  Bottom 0.254: U1.28 11.03,42.17 v10.48,41.62
N$29  (via drill 0.35)
  Top 0.254: U6.41 20.3,17.17 v18.89,17.17 | v6.83,3.68 R16.2
  Bottom 0.254: v18.89,17.17 17.78,17.17 6.83,6.22 v6.83,3.68
N$30  (via drill 0.35)
  Top 0.254: R5.2 15.72,50.98 15.72,49.24 15.4,48.92 v15.08,48.92
  Bottom 0.254: U1.3 15.31,48.69 v15.08,48.92
N$31  (via drill 0.35)
  Top 0.254: v13.49,41.14 12.38,40.03 10.64,40.03 9.53,38.92 9.53,37.65 8.1,36.22 8.1,32.73 8.57,32.25 10.16,32.25 10.48,31.93 10.48,29.71 11.59,28.6 11.59,25.43 12.06,24.95 12.86,24.95 13.18,25.27 13.18,25.58 13.49,25.9 13.97,25.9 | U6.1 17.48,22.39 16.35,23.52 15.56,23.52 15.08,24 15.08,25.58 14.76,25.9 13.97,25.9 | TP1.TP 13.97,25.9
  Bottom 0.254: U1.9 19.95,45.37 19.68,45.11 19.68,43.52 19.05,42.89 18.1,42.89 16.99,41.78 14.13,41.78 v13.49,41.14
N$32
  Bottom 0.254: U1.31 11.18,44.57 10.95,44.79 R4.2
N$33
  Top 0.254: LED2.A R16.1
N$34
  Bottom 0.254: R21.1 6.51,12.57 8.73,12.57 8.9,12.39 U5.4 9.42,11.98 9.68,12.25 9.68,14.31 10,14.63 10.01,14.62 SIM1.C7
N$35  (via drill 0.35)
  Top 0.406: U$1.VBUS 4.75,28.3 5.4,27.65 v5.4,26.7
  Bottom 0.254: R1.2 v5.4,26.7
  Bottom 0.406: C1.1 v5.4,26.7
  Bottom 0.508: U4.4 C1.1
N$36  (via drill 0.35)
  Top 0.254: U7.7 19.66,46.72 19.37,47.02 18.89,47.02 18.41,46.54 v18.41,45.27 17.62,44.47 17.62,43.68 18.1,43.2 19.21,43.2 R8.1
  Bottom 0.254: U1.30 13.09,43.77 13.65,43.2 16.51,43.2 18.41,45.11 v18.41,45.27
N$37  (via drill 0.35)
  Top 0.254: v18.41,44 20,44 R7.1 19.16,45.16 U7.6
  Bottom 0.254: U1.29 13.25,42.97 13.49,42.73 16.67,42.73 17.94,44 v18.41,44
N$38  (via drill 0.35)
  Top 0.254: 14.61,50.5 R6.2 14.13,50.03 v14.13,48.92
  Bottom 0.254: U1.2 14.51,48.54 v14.13,48.92
N$39
  Top 0.406: U6.28 11.98,3.28 C21.1
N$40  (via drill 0.35)
  Top 0.254: v15.88,37.01 16.99,37.01 17.3,37.33 19.53,37.33 v20.16,36.7 | v20,25.9 20,24.79 R17.1
  Bottom 0.254: v20.16,36.7 19.05,35.59 19.05,28.28 R18.1 19.36,27.02 20,26.38 v20,25.9 | U1.21 16.11,37.25 v15.88,37.01
N$41  (via drill 0.35)
  Top 0.254: LED1.C 12.54,28.44 11.91,29.08 v11.91,29.87
  Bottom 0.254: U4.1 11.74,30.03 v11.91,29.87
N$42  (via drill 0.35)
  Top 0.254: v10.79,38.6 11.27,39.08 13.02,39.08 13.34,38.76 13.34,38.28 15.4,36.22 | C13.1 17.94,31.46 21.59,31.46 23.5,33.36 C12.+
  Top 0.406: U3.23 14.79,35.61 15.4,36.22 C11.1 19.53,36.22 20,35.74 22.23,35.74 C12.+
  Bottom 0.254: v10.79,38.6 10.48,38.92 10.48,39.71 10.16,40.03 7.62,40.03 7.46,39.87 R10.2 R9.2
  Bottom 0.406: Q1.3 22.75,32.62 23.5,33.36 C12.+
N$44  (via drill 0.35)
  Top 0.254: U6.39 19.22,14.94 18.73,15.42 18.73,16.06 18.26,16.54 18.26,17.8 18.73,18.28 18.73,18.76 19.53,19.55 19.53,21.14 19.05,21.62 v19.05,26.06
  Bottom 0.254: 18.57,26.54 v19.05,26.06 18.41,26.7 18.41,29.08 18.57,29.23 18.57,36.06 18.51,36.12 U1.18
N$47
  Top 0.254: LED3.A R5.1
N$48
  Top 0.254: R14.2 9.53,30.03 11.11,28.44 11.11,25.27 11.91,24.47 13.65,24.47 R15.2 14.13,24.16 15.24,23.04 15.72,23.04 16.38,22.38 U6.2 16.35,21.82
N$49
  Top 0.254: LED4.A R6.1
N$50  (via drill 0.35)
  Top 0.254: v24.77,18.44 25.86,19.54 25.86,19.71 | 25.86,19.71 Q2.1 | v20.8,21.3 20.16,21.93 R17.2 | C15.2 26.51,15.74 26.51,19.06 25.86,19.71
  Bottom 0.254: v24.77,18.44 23.65,18.44 v20.8,21.3
N$53  (via drill 0.35)
  Top 0.254: v15.24,39.55 15.24,38.6 16.03,37.81 20,37.81 21.43,36.38 22.54,36.38 23.18,35.74 23.97,35.74 24.77,34.95 24.77,34 20.87,30.11 20.56,30.11 | R12.1 19.21,30.19 20.48,30.19 20.56,30.11 | 20.56,30.11 R11.1
  Bottom 0.254: U1.15 19.91,40.57 19.68,40.35 19.68,39.87 19.05,39.24 16.35,39.24 16.03,39.55 v15.24,39.55
N$54  (via drill 0.35)
  Top 0.254: R12.2 19.05,28.6 | R12.2 C13.2 | R12.2 19.21,28.6 19.53,28.92 21.75,28.92 22.07,29.23 22.07,30.66 22.54,31.14 v23.02,31.14
  Bottom 0.254: 22.02,30.35 Q1.1 22.5,30.62 v23.02,31.14
N$56  (via drill 0.35)
  Top 0.254: U6.16 6.35,14.94 6.68,14.94 7.31,14.94 7.94,14.31 7.94,12.41 v6.83,11.3
  Bottom 0.254: R20.2 3.97,11.3 4.13,11.14 5.87,11.14 6.03,11.3 v6.83,11.3
N$57  (via drill 0.35)
  Top 0.254: v6.51,18.12 6.51,16.85 6.83,16.54 6.83,16.06 8.41,14.47 8.41,12.25 7.62,11.46 7.62,11.14 7.14,10.66 6.51,10.66 6.19,10.98 6.19,12.41 6.83,13.04 6.99,13.04 7.46,13.52 7.46,14.15 7.14,14.47 6.35,14.47 5.71,13.84 U6.17
  Bottom 0.254: R19.2 4.13,19.07 5.56,19.07 v6.51,18.12
VBAT
  Top 1.016: Q2.2 23.66,20.04 25.77,22.14 P1.1
  Bottom 0.254: Q3.4 24.14,40.4 25.4,39.14 25.4,33.04 25.88,32.57 25.88,30.35 26.72,29.51 U2.3 | R18.2 14.6,27.96 14.37,27.73 C2.1
  Bottom 0.406: P1.1 26.83,24.58 C3.1 26.83,28.33 U2.3
  Bottom 0.508: U4.3 12.7,28.13 13.18,27.65 C2.1 | 16.83,26.38 | 16.83,26.38 16.83,25.58 18.57,23.84 21.75,23.84 22.54,24.63 24.65,24.63 P1.1 | 16.83,26.38 16.03,27.17 14.92,27.17 14.37,27.73

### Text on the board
tPlace: GPS | GND | SWC | SWD | RST | TX | RX | GND | SafeBee.gr | - | + | GSM
bPlace: 190208 1.3 | zakkemble.net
